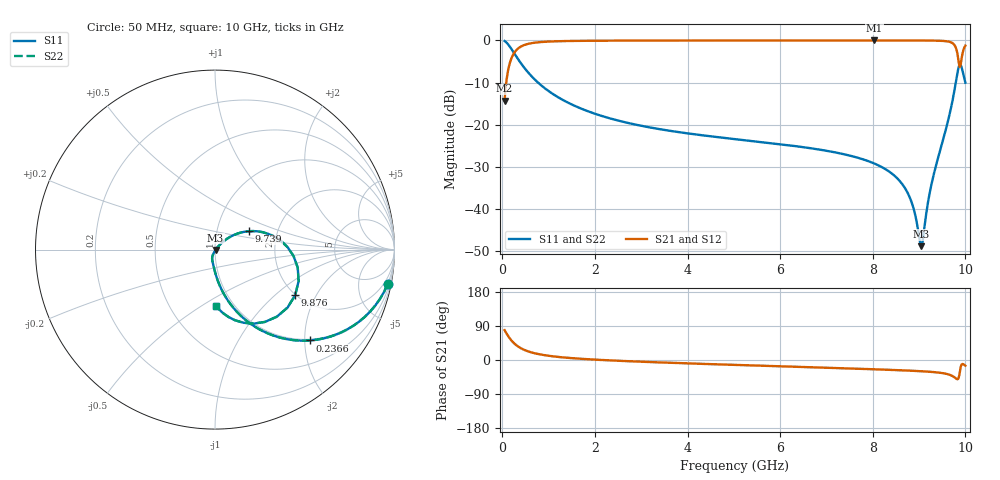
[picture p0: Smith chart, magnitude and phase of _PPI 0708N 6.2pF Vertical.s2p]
! S-Parameter data specifications (vertical orientation):
! Substrate: 40-mil Rogers 3003C, Substrate thickness, H=1.016mm, Dielectric constant, Er=3, Conductor thickness, T_mtl=0.043mm, Loss Tangent, Tand=0.003
! PCB Mounting Pad Footprint: Pad width, PadW=2.54mm , Pad length, PadL=0.51mm , Pad gap, PadG (edge-to-edge)=0.71mm , Reference planes=1.73mm apart
! Created Tue Jan 16 08:46:07 2018
# GHz S MA R 50
! 2 Port Network Data from SP1.SP block
! freq  magS11  angS11  magS21  angS21  magS12  angS12  magS22  angS22
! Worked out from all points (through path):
!   801 points, 50 MHz to 10 GHz, reference 50 ohm
!   highest |S21| = -0.02 dB at 8.035 GHz (marker M1); lowest = -14.3 dB at 50 MHz (marker M2)
!   group delay of S21, straight-line fit = 15.8 ps
!   lowest |S11| = -48.8 dB at 9.042 GHz (marker M3), VSWR 1.01, Z = 50.3 - j0.233 ohm
!   |S11| at or under -10 dB: 771.1 MHz to 9.792 GHz (9.021 GHz wide, 171 % of centre); 9.998982 GHz to end of sweep
!   |S22| runs from -48.8 to -0.2 dB; largest |S21 - S12| = 0
!   S11 on the Smith chart (normalised r, x): 50 MHz: 1, -10; 236.6 MHz: 0.97, -2.12; 9.739 GHz: 1.43, +0.31; 9.876 GHz: 1.99, -1.37; 10 GHz: 0.83, -0.58
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0.05  0.9812 -11.3  0.1929 78.7  0.1929 78.7  0.9812 -11.3
0.1495  0.8621 -30.9  0.5066 59.0  0.5066 59.0  0.8621 -30.9
0.2365625  0.7324 -43.7  0.6806 46.3  0.6806 46.3  0.7324 -43.7
0.4106875  0.5275 -59.5  0.8492 30.4  0.8492 30.4  0.5275 -59.5
0.6594375  0.3622 -70.9  0.9317 19.0  0.9317 19.0  0.3622 -70.9
1.716625  0.1542 -86.7  0.9874 3.1  0.9874 3.1  0.1542 -86.7
3.370812  0.08914 -95.7  0.9951 -6.2  0.9951 -6.2  0.08914 -95.7
5.025  0.06754 -102.1  0.9965 -12.9  0.9965 -12.9  0.06754 -102.1
6.691625  0.05234 -107.8  0.9971 -19.2  0.9971 -19.2  0.05234 -107.8
8.034875  0.03468 -111.6  0.9973 -24.5  0.9973 -24.5  0.03468 -111.6
8.345812  0.02806 -111.8  0.9973 -25.9  0.9973 -25.9  0.02806 -111.8
8.768688  0.01496 -107.9  0.9969 -27.9  0.9969 -27.9  0.01496 -107.9
8.880625  0.01019 -101.9  0.9967 -28.6  0.9967 -28.6  0.01019 -101.9
9.042312  0.003636 -39.7  0.996 -29.6  0.996 -29.6  0.003636 -39.7
9.092063  0.004785 6.1  0.9957 -29.9  0.9957 -29.9  0.004785 6.1
9.278625  0.02095 42.9  0.9938 -31.5  0.9938 -31.5  0.02095 42.9
9.589562  0.09308 41.7  0.9765 -36.5  0.9765 -36.5  0.09308 41.7
9.738812  0.2157 28.4  0.9117 -43.6  0.9117 -43.6  0.2157 28.4
9.801  0.3372 12.6  0.7953 -49.3  0.7953 -49.3  0.3372 12.6
9.875625  0.5138 -29.6  0.4868 -34.9  0.4868 -34.9  0.5138 -29.6
9.925375  0.465 -62.5  0.6414 -11.0  0.6414 -11.0  0.465 -62.5
10  0.3146 -88.9  0.8656 -15.0  0.8656 -15.0  0.3146 -88.9
